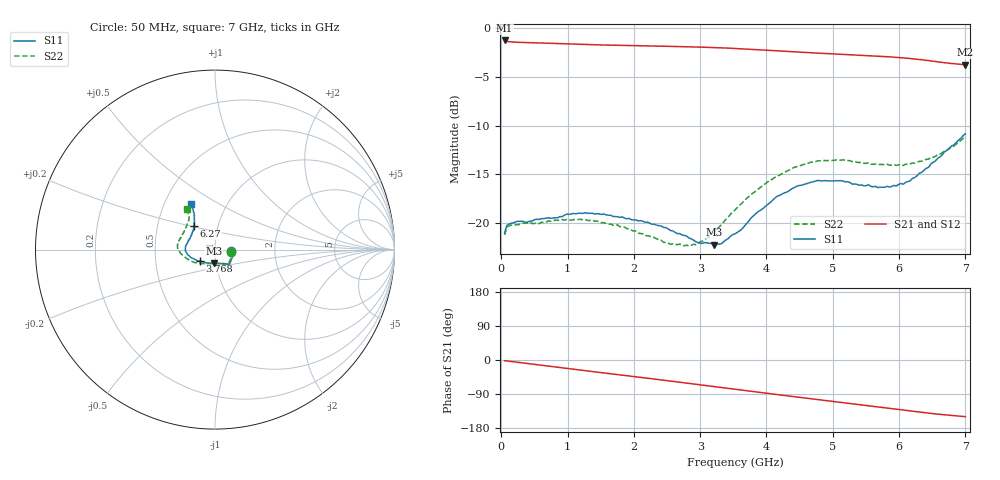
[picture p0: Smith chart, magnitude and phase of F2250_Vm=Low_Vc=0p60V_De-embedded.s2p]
! Integrated Device Technology
! Corporate Headquarters
! 6024 Silver Creek Valley Road
! San Jose, CA 95138  USA
! Phone:  1-408-284-8200
! Toll Free:  1-800-223-1366
! Webpage:  http://www.idt.com/
! Timing and RF Division
! 515 Groton Road, Suite 102
! Westford, MA 01886-6024
! Device:  F2250
! Description: Voltage Variable RF Attenuator
! Frequency:  50.0 -  6000.00 MHz
! Package:  3x3 mm Thin QFN Plastic Package: 16 pin
! Ports:  2 RF, 3 DC
!  Pin  1  = GND
!  Pin  2  = NC
!  Pin  3  = RF1  = Port 1
!  Pin  4  = NC
!  Pin  5  = GND
!  Pin  6  = GND
!  Pin  7  = GND
!  Pin  8  = GND
!  Pin  9  = NC
!  Pin 10  = RF2  = Port 2
!  Pin 11  = NC
!  Pin 12  = GND
!  Pin 13  = GND
!  Pin 14  = VCNTRL
!  Pin 15  = VDD
!  Pin 16  = VMODE
! Vcntrl:  0.600 Volts
! Vmode:  +0.000 Volts
! Vdd:  +3.30  Volts
! Current:  1.136 mA
! Data:  The device was measured on a the F2250 evaluation board which has
!  individual transmission lines to the RF pins.  Data was collected
!  using a calibrated network analyzer.  The evaluation board was
!  de-embedded using a TRL calibration technique.
!  The reference plane is the edge of the package pin.
! Misc:  SN 10
!  Action Tracker AT0258
! Date Measured:  2014-11-26
! Date:  2015-10-15  MJV
! Note:
!  Integrated Device Technology supplies this data as a sample of measured
!  data at the package pin for this product.  Your particular data for this
!  product may vary.
!  Data was taken at 25 degrees C.
!  Integrated Device Technology reserves the right to change this data at anytime.
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# GHz S dB R 50
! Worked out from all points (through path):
!   201 points, 50 MHz to 7 GHz, reference 50 ohm
!   highest |S21| = -1.26 dB at 50 MHz (marker M1); lowest = -3.8 dB at 7 GHz (marker M2)
!   group delay of S21, straight-line fit = 60.1 ps
!   lowest |S11| = -22.2 dB at 3.212 GHz (marker M3), VSWR 1.17, Z = 48.7 - j7.58 ohm
!   |S11| at or under -10 dB: start of sweep to end of sweep
!   |S22| runs from -22.3 to -11.1 dB; largest |S21 - S12| = 0.00043
!   S11 on the Smith chart (normalised r, x): 50 MHz: 1.20, -0.02; 3.768 GHz: 0.84, -0.11; 6.27 GHz: 0.77, +0.21; 7 GHz: 0.68, +0.38
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0.05  -20.96 -6.1  -1.26 -1.8  -1.26 -1.8  -21.19 -7.2
0.08475  -20.20 -6.2  -1.36 -2.5  -1.35 -2.5  -20.40 -6.9
0.15425  -19.99 -8.3  -1.41 -4.0  -1.41 -4.0  -20.18 -8.8
0.6755  -19.49 -27.3  -1.54 -15.4  -1.54 -15.4  -19.88 -31.0
1.2315  -18.98 -44.1  -1.67 -27.4  -1.66 -27.4  -19.64 -52.5
1.75275  -19.33 -51.0  -1.76 -38.5  -1.76 -38.5  -20.17 -62.4
2.37825  -20.24 -53.9  -1.85 -51.8  -1.85 -51.8  -21.68 -71.4
2.83  -21.51 -67.2  -1.92 -61.7  -1.91 -61.7  -22.35 -92.5
3.0385  -22.04 -81.2  -1.95 -66.3  -1.95 -66.3  -21.83 -107.5
3.21225  -22.19 -95.2  -1.99 -70.2  -1.99 -70.2  -20.87 -120.2
3.3165  -22.11 -106.0  -2.02 -72.5  -2.02 -72.5  -20.18 -127.1
3.525  -21.09 -124.1  -2.08 -77.2  -2.08 -77.2  -18.64 -139.2
3.76825  -19.46 -142.2  -2.17 -82.6  -2.17 -82.6  -17.04 -150.7
4.1505  -17.28 -159.7  -2.32 -91.0  -2.32 -91.0  -15.21 -166.4
4.46325  -16.18 -169.6  -2.44 -97.7  -2.44 -97.8  -14.18 -175.3
4.7065  -15.74 -176.3  -2.54 -103.0  -2.54 -103.0  -13.73 179.2
5.15825  -15.68 172.6  -2.70 -112.7  -2.70 -112.7  -13.50 169.4
5.85325  -16.29 148.6  -2.94 -127.6  -2.94 -127.6  -14.05 153.4
6.06175  -16.00 140.3  -3.05 -132.1  -3.05 -132.1  -14.08 147.4
6.27025  -15.14 131.9  -3.19 -136.7  -3.19 -136.7  -13.77 140.8
6.61775  -13.20 121.4  -3.49 -143.4  -3.49 -143.4  -12.91 129.2
7  -10.84 117.6  -3.75 -149.5  -3.76 -149.6  -11.14 124.9
